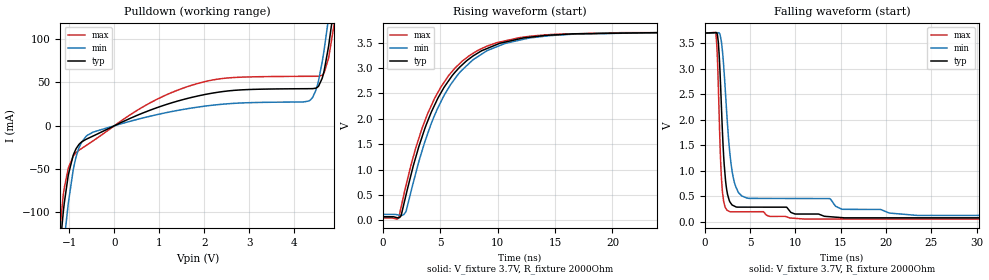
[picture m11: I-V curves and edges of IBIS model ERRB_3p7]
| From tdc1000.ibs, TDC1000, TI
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|   Model
[Model]   ERRB_3p7
Model_type   Open_drain
Polarity   Non-Inverting
Vmeas = 1.85
Vref = 3.7
Cref = 1pF
Rref = 2000
|   typ   min   max
C_comp   0.791pF   0.756pF   0.854pF
[Voltage Range]   3.7   3.699   3.701
[Temperature Range]   27   125   -40
[Pullup Reference]   3.7   3.699   3.701
[Pulldown Reference]   0   0   0
[Power Clamp Reference]   3.7   3.699   3.701
[GND Clamp Reference]   0   0   0
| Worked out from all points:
|   slope of the pulldown table from 0 to 0.555 V, typ, clamps not added: 42.5 ohm
|   falling waveform, V_fixture 3.7V, R_fixture 2000Ohm: 20-80 % time 623ps typ, 1.07ns min, 428ps max; typ from 3.7 V to 0.072 V
|   rising waveform, V_fixture 3.7V, R_fixture 2000Ohm: 20-80 % time 4.17ns typ, 4.24ns min, 4.06ns max; typ from 0.072 V to 3.7 V
[Pulldown]
|   Voltage   I(typ)   I(min)   I(max)
-3.7V     -1.758A    -1.795A    -1.732A
-1.38V    -235mA     -282.1mA   -207.9mA
-1.114V   -88.89mA   -131.1mA   -71.45mA
-1.025V   -56.65mA   -89.3mA    -48.81mA
-847.3mV  -26.08mA   -34.96mA   -30.75mA
-481mV    -12.03mA   -7.523mA   -17.68mA
1.728V    32.82mA    20.52mA    46.86mA
4.336V    42.78mA    28.83mA    57.07mA
4.625V    54.66mA    73.29mA    58.2mA
4.769V    91.89mA    124.7mA    78.21mA
4.914V    146.7mA    186.2mA    124.1mA
7.4V      1.445A     1.512A     1.385A
[Ramp]
R_load = 2000
|   typ   min   max
dV/dt_r   2.17668/4.17173e-09   2.14829/4.22421e-09   2.19149/4.05983e-09
dV/dt_f   2.17668/6.23322e-10   2.14829/1.06349e-09   2.19149/4.25484e-10
[Falling Waveform]
V_fixture = 3.7V
V_fixture_min = 3.699V
V_fixture_max = 3.701V
R_fixture = 2000Ohm
C_fixture = 0F
|   Time   V(typ)   V(min)   V(max)
0s        3.7V       3.699V     3.701V
1.17ns    3.709V     3.706V     3.712V
1.382ns   3.676V     3.707V     3.218V
1.902ns   1.926V     3.412V     668.9mV
2.286ns   798.5mV    2.495V     266.2mV
2.758ns   386.9mV    1.342V     193mV
3.351ns   294.6mV    710.9mV    190.8mV
4.645ns   282.4mV    461.3mV    191.7mV
23.44ns   72.59mV    119.7mV    48.78mV
100ns     72.19mV    118.5mV    48.51mV
[Rising Waveform]
V_fixture = 3.7V
V_fixture_min = 3.699V
V_fixture_max = 3.701V
R_fixture = 2000Ohm
C_fixture = 0F
|   Time   V(typ)   V(min)   V(max)
0s        72.19mV    118.5mV    48.51mV
1.405ns   52.63mV    105.7mV    57.68mV
1.608ns   95.29mV    96.72mV    264.6mV
1.999ns   468.6mV    163.1mV    657.9mV
3.736ns   1.849V     1.59V      1.996V
5.703ns   2.738V     2.596V     2.839V
7.846ns   3.235V     3.16V      3.287V
11.92ns   3.577V     3.55V      3.599V
22.97ns   3.695V     3.695V     3.697V
100ns     3.7V       3.699V     3.701V
